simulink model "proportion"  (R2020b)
settings: Solver=FixedStepAuto  StartTime=0.0  StopTime=10  FixedStep=0.02  RelTol=1e-3
libraries: sldrtlib x1

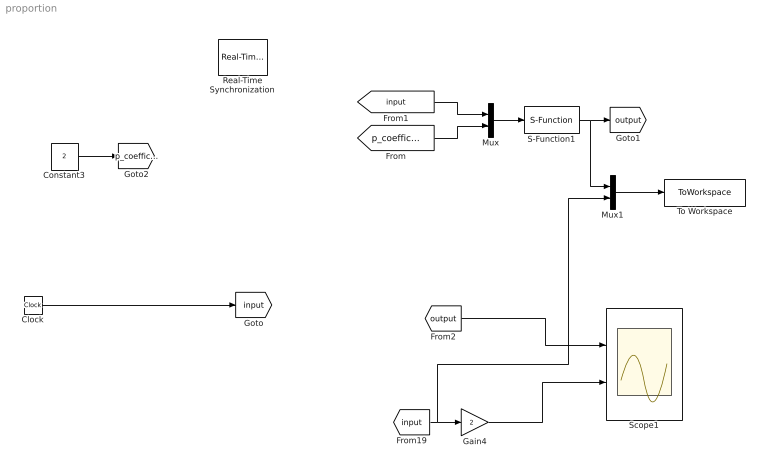
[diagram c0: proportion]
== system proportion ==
  Clock : Clock
  Constant3 : Constant  Value=2
  Gain4 : Gain  Gain=2
  Mux : Mux  Inputs=2
  Mux1 : Mux  Inputs=2
  Real-Time Synchronization : sldrtlib/Real-Time Synchronization  SampleTime=0.02  MaxMissedTicks=inf  ShowMissedTicks=off  YieldWhenWaiting=off
  S-Function1 : S-Function  FunctionName=modbusComproportion  SFunctionDeploymentMode=off  EnableBusSupport=off
  Scope1 : Scope  NumInputPorts=2
  To Workspace : ToWorkspace  VariableName=simout  SampleTime=-1
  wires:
  Clock/1 -> [input]
  [input] -> Mux1/2, Gain4/1
  S-Function1/1 -> Mux1/1, [output]
  [output] -> Scope1/1
  Gain4/1 -> Scope1/2
  [input] -> Mux/1
  [p_coefficient] -> Mux/2
  Mux/1 -> S-Function1/1
  Constant3/1 -> [p_coefficient]
  Mux1/1 -> To Workspace/1
